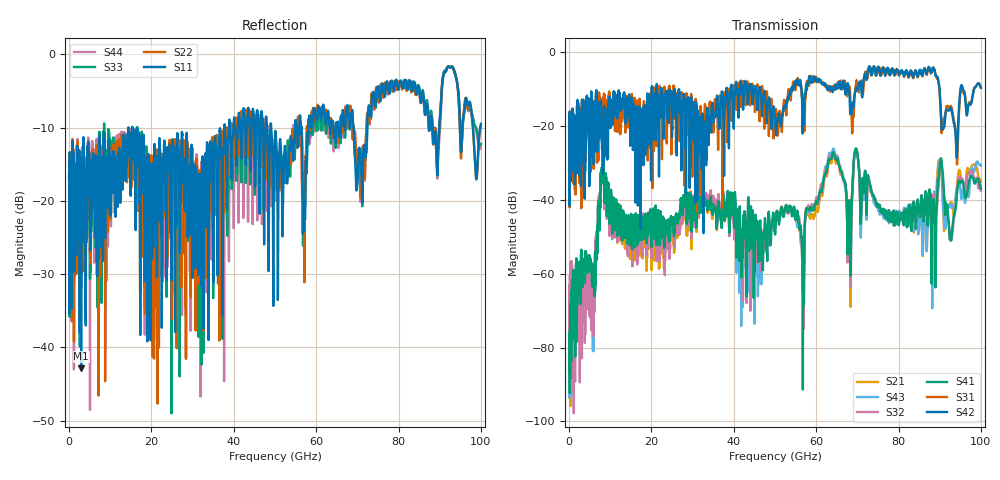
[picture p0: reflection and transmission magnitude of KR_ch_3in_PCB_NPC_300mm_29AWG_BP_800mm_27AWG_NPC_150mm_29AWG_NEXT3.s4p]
# GHz S RI R 45
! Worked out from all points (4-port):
!   4000 points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, 25 MHz to 100 GHz, reference 45 ohm
!   strongest paths, dB at 25 MHz, 25.02 GHz, 50.02 GHz, 75.03 GHz, 100 GHz:
!     S42: -21.2, -20.7, -18.6, -4.1, -9.8
!     S31: -21.2, -12.7, -15.8, -5.0, -9.6
!     S41: -86.3, -46.1, -49.4, -41.4, -37.0
!     S32: -85.6, -48.2, -47.3, -41.4, -37.5
!     S43: -89.3, -48.2, -46.3, -42.3, -30.8
!     S21: -93.5, -50.7, -47.2, -42.2, -35.2
!   lowest |S11| = -42.9 dB at 2.95 GHz (marker M1), VSWR 1.01, Z = 45.6 - j0.1 ohm
!   |S11| at or under -10 dB: start of sweep to 14.45 GHz; 15.35 GHz to 37.72 GHz (22.36 GHz wide, 84.3 % of centre); 49.09 GHz to 54.88 GHz (5.797 GHz wide, 11.2 % of centre)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
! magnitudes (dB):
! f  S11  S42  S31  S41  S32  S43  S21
! 25 MHz  -16.5  -21.2  -21.2  -86.3  -85.6  -89.3  -93.5
! 2.95 GHz  -42.9  -17.0  -20.1  -63.4  -61.6  -67.6  -65.9
! 5.85 GHz  -14.4  -13.3  -15.4  -59.9  -67.9  -70.9  -73.6
! 8.075 GHz  -16.5  -20.2  -20.6  -35.3  -35.4  -35.3  -35.6
! 56.67 GHz  -17.3  -19.7  -13.6  -56.7  -56.3  -60.7  -59.3
! 63.88 GHz  -9.3  -10.0  -9.5  -28.3  -28.3  -27.3  -29.0
! 100 GHz  -9.5  -9.8  -9.6  -37.0  -37.5  -30.8  -35.2
